[IBIS Ver]   4.1
[File Name]   sprm792.ibs
[File Rev]   1.0
[Date]   October 18, 2021
[Source]   File originated at Texas Instruments
[Copyright]   (c) 2012, Texas Instruments Inc.
[Component]   f771860xpmq
[Manufacturer] Texas Instruments
[Package]
| Variable   Typ   Min   Max
R_pkg   0.200   0.073   0.251
L_pkg   4.73E-9   3.87E-09   5.45E-09
C_pkg   4.26E-13   3.54E-13   5.21E-13
[Pin]   signal_name   model_name   R_pin   L_pin   C_pin
1   GPIO29   BCPF335585DSHYPBFZ   2.35E-01   5.23E-09   3.69E-13
2   GPIO28   BCF3385DSHYPBFZ_USF   2.23E-01   5.01E-09   4.49E-13
3   XRSN   BQ0491FS_USF   2.11E-01   4.76E-09   4.25E-13
4   VDD   NC   2.17E-01   4.79E-09   4.05E-13
5   VSS   NC   2.11E-01   4.69E-09   3.85E-13
6   A6   ICF33SHYPB_USF   2.41E-01   5.08E-09   4.02E-13
7   B2/C6   ICF33SHYPB_USF   2.28E-01   4.83E-09   4.09E-13
8   A3/B3/VDAC,C5   ICF33SHYPB_USF   2.24E-01   4.74E-09   4.48E-13
9   A2/B6/C9   ICF33SHYPB_USF   2.08E-01   4.53E-09   3.68E-13
10   A15/B9/C7   ICF33SHYPB_USF   2.02E-01   4.47E-09   4.25E-13
11   A14/B14/C4   ICF33SHYPB_USF   2.00E-01   4.46E-09   3.86E-13
12   A11/B10/C0   ICF33SHYPB_USF   2.00E-01   4.50E-09   4.03E-13
13   A5/B12/C2   ICF33SHYPB_USF   2.03E-01   4.60E-09   4.65E-13
14   A1/B7/DACB_OUT   ICF33SHYPB_USF   2.11E-01   4.76E-09   4.39E-13
15   A0/B15/C15/DACA_OUT   ICF33SHYPB_USF   2.23E-01   5.00E-09   4.58E-13
16   VREFHI   NC   7.85E-02   4.33E-09   4.34E-13
17   VREFLO   NC   7.84E-02   4.33E-09   4.38E-13
18   A12,C1   ICF33SHYPB_USF   2.27E-01   5.07E-09   5.03E-13
19   A7/C3   ICF33SHYPB_USF   2.20E-01   4.91E-09   4.34E-13
20   A8/B0/C11   ICF33SHYPB_USF   2.15E-01   4.77E-09   4.75E-13
21   VSSA   NC   7.16E-02   3.92E-09   5.03E-13
22   VDDA   NC   7.13E-02   3.87E-09   4.79E-13
23   A4/B8/C14   ICF33SHYPB_USF   2.12E-01   4.64E-09   4.33E-13
24   A9/B4/C8   ICF33SHYPB_USF   2.13E-01   4.65E-09   4.05E-13
25   A10/B1/C10   ICF33SHYPB_USF   2.21E-01   4.73E-09   3.57E-13
26   VSS   NC   1.10E-01   4.12E-09   4.30E-13
27   VDD   NC   1.12E-01   4.18E-09   4.55E-13
28   VDDIO   NC   2.20E-01   4.84E-09   4.54E-13
29   GPIO13   BCF3385DSHYPBFZ_USF   2.08E-01   4.64E-09   3.94E-13
30   GPIO12   BCF3385DSHYPBFZ_USF   2.08E-01   4.69E-09   4.20E-13
31   GPIO11   BCF3385DSHYPBFZ_USF   2.13E-01   4.84E-09   4.40E-13
32   GPIO33   BCPF335585DSHYPBFZ   2.34E-01   5.23E-09   3.71E-13
33   GPIO16   BCF3385DSHYPBFZ   2.36E-01   5.26E-09   3.79E-13
34   GPIO17   BCF3385DSHYPBFZ   2.18E-01   4.93E-09   4.44E-13
35   GPIO24   BCPF335585DSHYPBFZ   2.17E-01   4.85E-09   4.22E-13
36   TCK   BCF3355DSHYPBFZ_TMS_USF   2.26E-01   4.93E-09   4.20E-13
37   GPIO37/TDO   BCPF335585DSHYPBFZ   2.17E-01   4.77E-09   4.10E-13
38   TMS   BCF3355DSHYPBFZ_TMS_USF   2.11E-01   4.63E-09   3.95E-13
39   GPIO35/TDI   BCF3385DSHYPBFZ   2.08E-01   4.55E-09   3.85E-13
40   GPIO32   BCPF335585DSHYPBFZ   2.07E-01   4.53E-09   3.54E-13
41   GPIO18/X2   BCPF335585DSHYPBFZ   2.07E-01   4.54E-09   4.00E-13
42   GPIO19/X1   BCF3385DSHYPBFZ   2.06E-01   4.54E-09   4.54E-13
43   VDDIO   NC   2.15E-01   4.63E-09   4.92E-13
44   VDD   NC   1.08E-01   4.12E-09   4.91E-13
45   VSS   NC   1.06E-01   4.09E-09   5.09E-13
46   VREGENZ   IQ0440FS_VREGENZ_USF   2.01E-01   4.60E-09   4.28E-13
47   GPIO8   BCF3385DSHYPBFZ_USF   2.15E-01   4.88E-09   4.42E-13
48   GPIO4   BCF3385DSHYPBFZ_USF   2.40E-01   5.33E-09   3.84E-13
49   GPIO3   BCF3385DSHYPBFZ_USF   2.43E-01   5.36E-09   3.76E-13
50   GPIO2   BCF3385DSHYPBFZ   2.51E-01   5.45E-09   4.68E-13
51   GPIO1   BCPF335585DSHYPBFZ   2.37E-01   5.18E-09   4.60E-13
52   GPIO0   BCF3385DSHYPBFZ   2.26E-01   4.93E-09   4.31E-13
53   GPIO40   BCF3385DSHYPBFZ_USF   2.21E-01   4.84E-09   4.11E-13
54   GPIO23   BCF3385DSHYPBFZ_USF   2.15E-01   4.70E-09   4.03E-13
55   GPIO41   BCF3385DSHYPBFZ_USF   2.13E-01   4.64E-09   3.91E-13
56   GPIO22   BCF3385DSHYPBFZ_USF   2.14E-01   4.64E-09   3.66E-13
57   GPIO7   BCF3385DSHYPBFZ_USF   2.21E-01   4.72E-09   3.72E-13
58   VSS   NC   1.15E-01   4.25E-09   4.88E-13
59   VDD   NC   1.12E-01   4.26E-09   5.21E-13
60   VDDIO   NC   2.45E-01   5.02E-09   4.64E-13
61   GPIO5   BCF3385DSHYPBFZ_USF   2.25E-01   4.92E-09   4.26E-13
62   GPIO9   BCF3385DSHYPBFZ_USF   2.33E-01   5.08E-09   4.36E-13
63   GPIO10   BCF3385DSHYPBFZ_USF   2.37E-01   5.22E-09   4.43E-13
64   GPIO6   BCF3385DSHYPBFZ_USF   2.28E-01   5.12E-09   3.58E-13
| End of package information
|   Component IQ0440FS_VREGENZ_USF
[Component]   IQ0440FS_VREGENZ_USF
[Manufacturer]   Texas Instruments
[Package]
|  variable   typ   min   max
R_pkg   0   0   0
L_pkg   0   0   0
C_pkg   0   0   0
[Pin]   signal_name   model_name   R_pin   L_pin   C_pin
VSS   VSS   GND
VDDS   VDDS   POWER
PAD   PAD   IQ0440FS_VREGENZ_USF
[Model Selector] IQ0440FS_VREGENZ_USF
VREGENZ_WK_PD_ON_3P3  Cell operated at 3.3(nom)
|VREGENZ_WK_PD_ON_3P3; WEAK_PULLDOWN_ON
VREGENZ_WK_PD_OFF_3P3  Cell operated at 3.3(nom)
|   Component ICF33SHYPB_USF
[Component]   ICF33SHYPB_USF
[Manufacturer]   Texas Instruments
[Package]
|  variable   typ   min   max
R_pkg   0   0   0
L_pkg   0   0   0
C_pkg   0   0   0
[Pin]   signal_name   model_name   R_pin   L_pin   C_pin
VSS   VSS   GND
VDDS   VDDS   POWER
PAD   PAD   ICF33SHYPB_USF
[Model Selector] ICF33SHYPB_USF
ICF_WK_PUPD_OFF_3P3  Cell operated at 3.3(nom)
|ICF_WK_PUPD_OFF_3P3; WEAK_PULL_OFF
ICF_WK_PU_ON_3P3  Cell operated at 3.3(nom)
|ICF_WK_PU_ON_3P3; WEAK_PULLUP_ON
ICF_WK_PD_ON_3P3  Cell operated at 3.3(nom)
|   Component ICF33SHYPB_FS_SFII_CUS
[Component]   ICF33SHYPB_FS_SFII_CUS
[Manufacturer]   Texas Instruments
[Package]
|  variable   typ   min   max
R_pkg   0   0   0
L_pkg   0   0   0
C_pkg   0   0   0
[Pin]   signal_name   model_name   R_pin   L_pin   C_pin
VSS   VSS   GND
VDDS   VDDS   POWER
PAD   PAD   ICF33SHYPB_FS_SFII_CUS
[Model Selector] ICF33SHYPB_FS_SFII_CUS
CUS_WK_PUPD_OFF_3P3  Cell operated at 3.3(nom)
|CUS_WK_PUPD_OFF_3P3; WEAK_PULL_OFF
CUS_WK_PU_ON_3P3  Cell operated at 3.3(nom)
|CUS_WK_PU_ON_3P3; WEAK_PULLUP_ON
CUS_WK_PD_ON_3P3  Cell operated at 3.3(nom)
|   Component BT3308BT5FSHYPB_SFII
[Component]   BT3308BT5FSHYPB_SFII
[Manufacturer]   Texas Instruments
[Package]
|  variable   typ   min   max
R_pkg   0   0   0
L_pkg   0   0   0
C_pkg   0   0   0
[Pin]   signal_name   model_name   R_pin   L_pin   C_pin
VSS   VSS   GND
VDDS   VDDS   POWER
PAD   PAD   BT3308BT5FSHYPB_SFII
[Model Selector] BT3308BT5FSHYPB_SFII
BT_OPEN_DRAIN_6MA_3P3  Cell operated at 3.3(nom)
|BT_OPEN_DRAIN_6MA_3P3
BT_WEAK_PD_ON_3P3  Cell operated at 3.3(nom)
|BT_WEAK_PD_ON_3P3
BT_OPEN_DRAIN_3MA_3P3  Cell operated at 3.3(nom)
|BT_OPEN_DRAIN_3MA_3P3
BT_DRIVER_MODE_6MA_3P3  Cell operated at 3.3(nom)
|BT_DRIVER_MODE_6MA_3P3
BT_DRIVER_MODE_3MA_3P3  Cell operated at 3.3(nom)
|BT_DRIVER_MODE_3MA_3P3
BT_WEAK_PU_ON_3P3  Cell operated at 3.3(nom)
|   Component BQ0491FS_USF
[Component]   BQ0491FS_USF
[Manufacturer]   Texas Instruments
[Package]
|  variable   typ   min   max
R_pkg   0   0   0
L_pkg   0   0   0
C_pkg   0   0   0
[Pin]   signal_name   model_name   R_pin   L_pin   C_pin
VSS   VSS   GND
VDDS   VDDS   POWER
PAD   PAD   BQ0491FS_USF
[Model Selector] BQ0491FS_USF
XRSN_WK_PU_ON_3P3  Cell operated at 3.3(nom)
|XRSN_WK_PU_ON_3P3; WEAK_PULLUP_ON
XRSN_OPEN_DRAIN  Cell operated at 3.3(nom)
|   Component BCPF335585DSHYPBFZ
[Component]   BCPF335585DSHYPBFZ
[Manufacturer]   Texas Instruments
[Package]
|  variable   typ   min   max
R_pkg   0   0   0
L_pkg   0   0   0
C_pkg   0   0   0
[Pin]   signal_name   model_name   R_pin   L_pin   C_pin
VSS   VSS   GND
VDDS   VDDS   POWER
PAD   PAD   BCPF335585DSHYPBFZ
[Model Selector] BCPF335585DSHYPBFZ
BCPF_WK_PU_ON_3P3  Cell operated at 3.3(nom)
|BCPF_WK_PU_ON_3P3; WEAK_PULLUP_ON
BCPF_DRIVER_4MA_3P3  Cell operated at 3.3(nom)
|BCPF_DRIVER_4MA_3P3
BCPF_DRIVER_2MA_3P3  Cell operated at 3.3(nom)
|BCPF_DRIVER_2MA_3P3
BCPF_WK_PD_ON_3P3  Cell operated at 3.3(nom)
|   Component BCF3385DSHYPBFZ_USF
[Component]   BCF3385DSHYPBFZ_USF
[Manufacturer]   Texas Instruments
[Package]
|  variable   typ   min   max
R_pkg   0   0   0
L_pkg   0   0   0
C_pkg   0   0   0
[Pin]   signal_name   model_name   R_pin   L_pin   C_pin
VSS   VSS   GND
VDDS   VDDS   POWER
PAD   PAD   BCF3385DSHYPBFZ_USF
[Model Selector] BCF3385DSHYPBFZ_USF
BCF3385DUSF_WK_PU  Cell operated at 3.3(nom)
| BCF3385DUSF_WK_PU; WEAK_PULLUP_ON
BCF3385DUSF_DRIVER_3P3  Cell operated at 3.3(nom)
|BCF3385DUSF_DRIVER_3P3
BCF3385DUSF_WK_PD  Cell operated at 3.3(nom)
|   Component BCF3385DSHYPBFZ
[Component]   BCF3385DSHYPBFZ
[Manufacturer]   Texas Instruments
[Package]
|  variable   typ   min   max
R_pkg   0   0   0
L_pkg   0   0   0
C_pkg   0   0   0
[Pin]   signal_name   model_name   R_pin   L_pin   C_pin
VSS   VSS   GND
VDDS   VDDS   POWER
PAD   PAD   BCF3385DSHYPBFZ
[Model Selector] BCF3385DSHYPBFZ
BCF3385D_WK_PU_3P3  Cell operated at 3.3(nom)
|BCF3385D_WK_PU_3P3; WEAK_PULLUP_ON
BCF3385D_DRIVER_3P3  Cell operated at 3.3(nom)
|BCF3385D_DRIVER_3P3
BCF3385D_WK_PD_3P3  Cell operated at 3.3(nom)
|   Component BCF3355DSHYPBFZ_TMS_USF
[Component]   BCF3355DSHYPBFZ_TMS_USF
[Manufacturer]   Texas Instruments
[Package]
|  variable   typ   min   max
R_pkg   0   0   0
L_pkg   0   0   0
C_pkg   0   0   0
[Pin]   signal_name   model_name   R_pin   L_pin   C_pin
VSS   VSS   GND
VDDS   VDDS   POWER
PAD   PAD   BCF3355DSHYPBFZ_TMS_USF
[Model Selector] BCF3355DSHYPBFZ_TMS_USF
TMS_WK_PU_ON_3P3  Cell operated at 3.3(nom)
|TMS_WK_PU_ON_3P3; WEAK_PULLUP_ON
TMS_DRIVER_3P3  Cell operated at 3.3(nom)
|TMS_DRIVER_3P3
TMS_WK_PD_ON_3P3  Cell operated at 3.3(nom)
|   Component BCF3335DSHYPBFZ
[Component]   BCF3335DSHYPBFZ
[Manufacturer]   Texas Instruments
[Package]
|  variable   typ   min   max
R_pkg   0   0   0
L_pkg   0   0   0
C_pkg   0   0   0
[Pin]   signal_name   model_name   R_pin   L_pin   C_pin
VSS   VSS   GND
VDDS   VDDS   POWER
PAD   PAD   BCF3335DSHYPBFZ
[Model Selector] BCF3335DSHYPBFZ
BCF3335D_WK_PU_3P3  Cell operated at 3.3(nom)
|BCF3335D_WK_PU_3P3; WEAK_PULLUP_ON
BCF3335D_DRIVER_3P3  Cell operated at 3.3(nom)
|BCF3335D_DRIVER_3P3
BCF3335D_WK_PD_3P3  Cell operated at 3.3(nom)
| Models and submodels in the file (32): VREGENZ_WK_PD_ON_3P3 (Input), VREGENZ_WK_PD_OFF_3P3 (Input), ICF_WK_PUPD_OFF_3P3 (Input), ICF_WK_PU_ON_3P3 (Input), ICF_WK_PD_ON_3P3 (Input), CUS_WK_PUPD_OFF_3P3 (Input), CUS_WK_PU_ON_3P3 (Input), CUS_WK_PD_ON_3P3 (Input), BT_OPEN_DRAIN_6MA_3P3 (I/O_open_drain), BT_WEAK_PD_ON_3P3 (Input), BT_OPEN_DRAIN_3MA_3P3 (I/O_open_drain), BT_DRIVER_MODE_6MA_3P3 (I/O), BT_DRIVER_MODE_3MA_3P3 (I/O), BT_WEAK_PU_ON_3P3 (Input), XRSN_WK_PU_ON_3P3 (Input), XRSN_OPEN_DRAIN (I/O_open_drain), BCPF_WK_PU_ON_3P3 (Input), BCPF_DRIVER_4MA_3P3 (I/O), BCPF_DRIVER_2MA_3P3 (I/O), BCPF_WK_PD_ON_3P3 (Input), BCF3385DUSF_WK_PU (Input), BCF3385DUSF_DRIVER_3P3 (I/O), BCF3385DUSF_WK_PD (Input), BCF3385D_WK_PU_3P3 (Input), BCF3385D_DRIVER_3P3 (I/O), BCF3385D_WK_PD_3P3 (Input), TMS_WK_PU_ON_3P3 (Input), TMS_DRIVER_3P3 (I/O), TMS_WK_PD_ON_3P3 (Input), BCF3335D_WK_PU_3P3 (Input), BCF3335D_DRIVER_3P3 (I/O), BCF3335D_WK_PD_3P3 (Input)
